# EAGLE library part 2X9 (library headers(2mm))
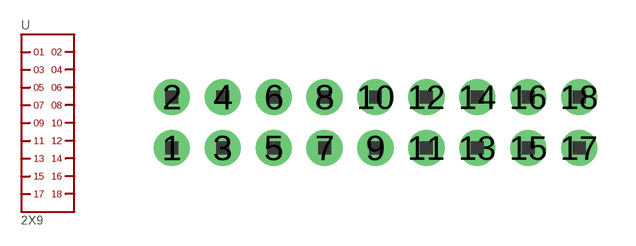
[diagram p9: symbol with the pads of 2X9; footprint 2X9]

Designator prefix -

## 2X9  [2X9]
1  1
2  2
3  3
4  4
5  5
6  6
7  7
8  8
9  9
10  10
11  11
12  12
13  13
14  14
15  15
16  16
17  17
18  18

## Footprint 2X9 (pad centres in mm)
drill 0.8 pad 1.422: 1 -8,-1; 2 -8,1; 3 -6,-1; 4 -6,1; 5 -4,-1; 6 -4,1; 7 -2,-1; 8 -2,1; 9 0,-1; 10 0,1; 11 2,-1; 12 2,1; 13 4,-1; 14 4,1; 15 6,-1; 16 6,1; 17 8,-1; 18 8,1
